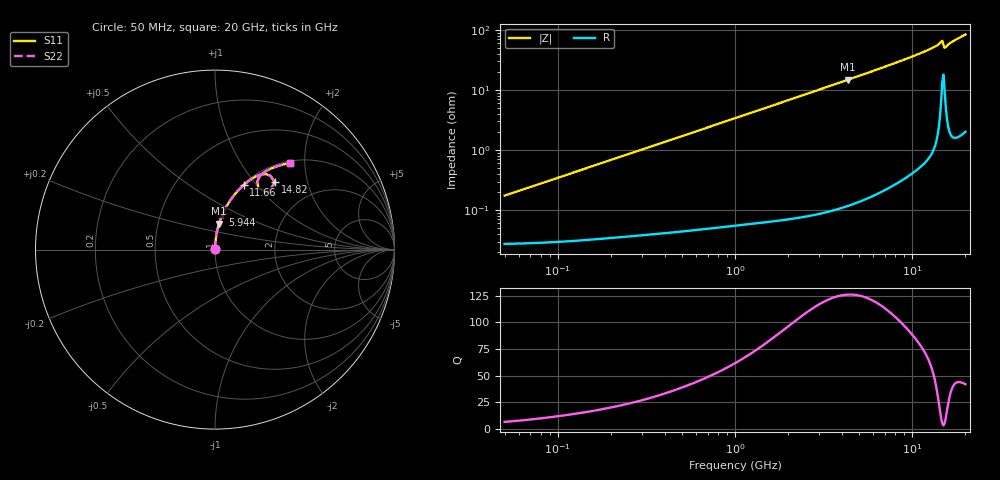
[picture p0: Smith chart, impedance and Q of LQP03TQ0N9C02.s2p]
!Murata Part Number: LQP03TQ0N9C02
!These Parameters are Measured in Series Mode Connection
!  o--[Z]--o
!Port1  Port2
!  o-------o
!Freq. Start=50[MHz] Stop=20[GHz], 401[Steps]
# Hz S RI R 50
!Freq.(Hz) S11(Real) S11(Imag) S21(Real) S21(Imag) S12(Real) S12(Imag) S22(Real) S22(Imag)
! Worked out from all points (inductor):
!   401 points, 50 MHz to 20 GHz, reference 50 ohm
!   read as one part in series: L = 551 pH near 51.52 MHz
!   highest Q = 126 at 4.34 GHz (marker M1), where L = 543 pH
!   S11 on the Smith chart (normalised r, x): 50 MHz: 1.00, +0.00; 5.944 GHz: 1.00, +0.41; 11.66 GHz: 1.01, +0.86; 14.82 GHz: 1.28, +1.28; 20 GHz: 1.04, +1.68
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5e7  0.000277 0.00173  0.9997 -0.00173  0.9997 -0.00173  0.000277 0.00173
1.364002e8  0.000336 0.00469  0.9997 -0.00469  0.9997 -0.00469  0.000336 0.00469
3.721004e8  0.000566 0.0127  0.9994 -0.0127  0.9994 -0.0127  0.000566 0.0127
1e9  0.0017 0.0338  0.9983 -0.0338  0.9983 -0.0338  0.0017 0.0338
1.714689e9  0.00401 0.0578  0.996 -0.0578  0.996 -0.0578  0.00401 0.0578
2.728004e9  0.00928 0.0916  0.9907 -0.0916  0.9907 -0.0916  0.00928 0.0916
4.34015e9  0.0226 0.1446  0.9774 -0.1446  0.9774 -0.1446  0.0226 0.1446
5.944466e9  0.0418 0.196  0.9582 -0.196  0.9582 -0.196  0.0418 0.196
7.442007e9  0.0652 0.2423  0.9348 -0.2423  0.9348 -0.2423  0.0652 0.2423
9.457416e9  0.1051 0.3013  0.8949 -0.3013  0.8949 -0.3013  0.1051 0.3013
1.166392e10  0.1609 0.3607  0.8391 -0.3607  0.8391 -0.3607  0.1609 0.3607
1.314879e10  0.2097 0.3977  0.7903 -0.3977  0.7903 -0.3977  0.2097 0.3977
1.417136e10  0.2629 0.4197  0.7371 -0.4197  0.7371 -0.4197  0.2629 0.4197
1.438523e10  0.282 0.4205  0.718 -0.4205  0.718 -0.4205  0.282 0.4205
1.460232e10  0.3083 0.4121  0.6917 -0.4121  0.6917 -0.4121  0.3083 0.4121
1.482269e10  0.3338 0.375  0.6662 -0.375  0.6662 -0.375  0.3338 0.375
1.527346e10  0.2424 0.3415  0.7576 -0.3415  0.7576 -0.3415  0.2424 0.3415
1.550395e10  0.2357 0.378  0.7643 -0.378  0.7643 -0.378  0.2357 0.378
1.573793e10  0.2442 0.4005  0.7558 -0.4005  0.7558 -0.4005  0.2442 0.4005
1.621653e10  0.2663 0.4249  0.7337 -0.4249  0.7337 -0.4249  0.2663 0.4249
1.696185e10  0.298 0.4448  0.702 -0.4448  0.702 -0.4448  0.298 0.4448
2e10  0.4162 0.4811  0.5838 -0.4811  0.5838 -0.4811  0.4162 0.4811
